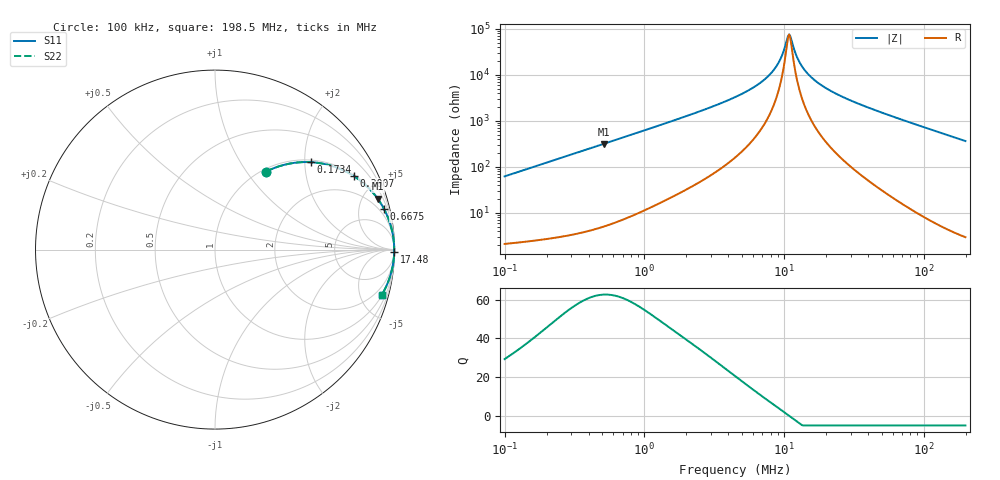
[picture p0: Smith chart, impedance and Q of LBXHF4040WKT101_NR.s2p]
! LBXHF4040WKT101_NR  S-PARAMETER MODEL  ( General Type )
! Model Generated by TAIYO YUDEN Corporation (http://www.ty-top.com)
! Version 1.0
! TAIYO YUDEN Control No. 210719NI43SB-FBB
! Copyright(c) 2021 TAIYO YUDEN CO.,LTD. All Rights Reserved.
! Product Description (link to TY-COMPAS)
! https://ds.yuden.co.jp/TYCOMPAS/or/detail?pn=LBXHF4040WKT101MNR&u=M
! Products Name : Inductors
! Characteristics :
!  Inductance : 100 uH , SRF(min) : 8.0 MHz , DC Resistance(max) : 1.512 Ohm
!  Rated Current : Saturation :460 mA , Temp Rise : 340 mA
!  Case Size : 4.0 x 4.0 / 0.157 x 0.157 [mm/inch] , Thickness : 2 / 0.079 [mm/inch]
!  (Conditions: Temperature = 25 degC , DC Bias Current/Voltage = 0A / 0V)
! External Node Assignments :
!  1  o---GGG---o  2
! GND o---------o GND
! Frequency Range : 0.1MHz  -  198.534594MHz  [ 402 STEP ]
# MHz S RI R 50
! Freq[MHz].  S11 Real  S11 Imag  S21 Real  S21 Imag  S12 Real  S12 Imag  S22 Real  S22 Imag
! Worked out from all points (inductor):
!   401 points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, 100 kHz to 198.5 MHz, reference 50 ohm
!   read as one part in series: L = 98.8 uH near 103.9 kHz
!   highest Q = 62.5 at 511.7 kHz (marker M1), where L = 98.4 uH
!   self-resonance near 10.87 MHz
!   S11 on the Smith chart (normalised r, x): 100 kHz: 1.04, +1.24; 173.4 kHz: 1.05, +2.15; 300.7 kHz: 1.07, +3.72; 667.5 kHz: 1.13, +8.26; 17.48 MHz: open; 198.5 MHz: 1.06, -7.28
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0.1  0.2859 0.4351  0.7141 -0.4351  0.7141 -0.4351  0.2859 0.4351
0.173418  0.5355 0.487  0.4645 -0.487  0.4645 -0.487  0.5355 0.487
0.300737  0.7718 0.4108  0.2282 -0.4108  0.2282 -0.4108  0.7718 0.4108
0.356769  0.8255 0.3712  0.1745 -0.3712  0.1745 -0.3712  0.8255 0.3712
0.511723  0.9055 0.2847  0.0945 -0.2847  0.0945 -0.2847  0.9055 0.2847
0.667512  0.9413 0.227  0.0587 -0.227  0.0587 -0.227  0.9413 0.227
1.272844  0.9819 0.1235  0.0181 -0.1235  0.0181 -0.1235  0.9819 0.1235
2.772065  0.9952 0.0548  0.00475 -0.0548  0.00475 -0.0548  0.9952 0.0548
4.541117  0.9976 0.0297  0.00237 -0.0297  0.00237 -0.0297  0.9976 0.0297
6.390948  0.9983 0.0167  0.00168 -0.0167  0.00168 -0.0167  0.9983 0.0167
8.026023  0.9986 0.00928  0.00145 -0.00928  0.00145 -0.00928  0.9986 0.00928
9.342371  0.9986 0.00459  0.00136 -0.00459  0.00136 -0.00459  0.9986 0.00459
10.46947  0.9987 0.00115  0.00134 -0.00115  0.00134 -0.00115  0.9987 0.00115
10.87461  0.9987 2.61e-06  0.00133 -2.61e-06  0.00133 -2.61e-06  0.9987 2.61e-06
11.29544  0.9987 -0.00114  0.00133 0.00114  0.00133 0.00114  0.9987 -0.00114
12.18657  0.9987 -0.00343  0.00134 0.00343  0.00134 0.00343  0.9987 -0.00343
13.148  0.9986 -0.00575  0.00135 0.00575  0.00135 0.00575  0.9986 -0.00575
15.89665  0.9985 -0.0117  0.00145 0.0117  0.00145 0.0117  0.9985 -0.0117
17.47948  0.9985 -0.0148  0.00153 0.0148  0.00153 0.0148  0.9985 -0.0148
27.04919  0.9977 -0.0314  0.0023 0.0314  0.0023 0.0314  0.9977 -0.0314
56.71438  0.9929 -0.0752  0.00706 0.0752  0.00706 0.0752  0.9929 -0.0752
198.5346  0.928 -0.2544  0.072 0.2544  0.072 0.2544  0.928 -0.2544
